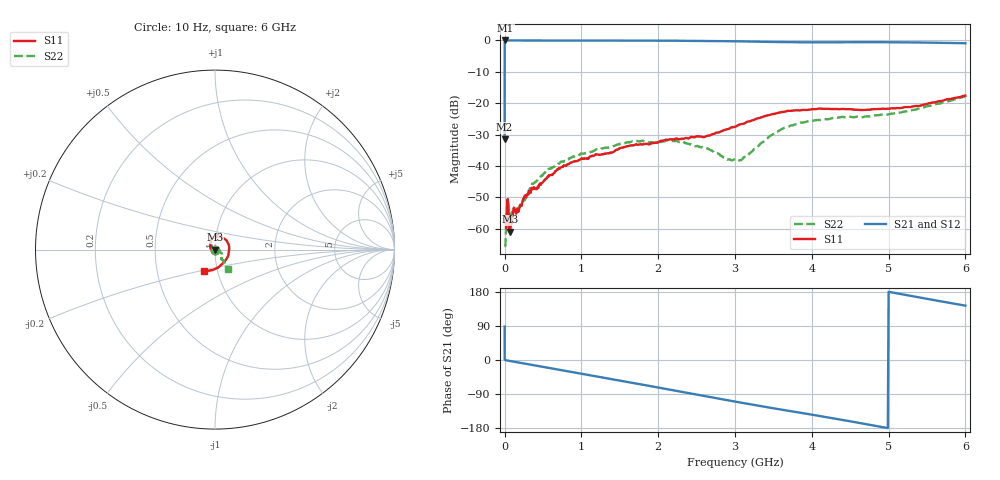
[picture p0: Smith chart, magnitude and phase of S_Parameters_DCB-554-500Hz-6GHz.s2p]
! MTS Systemtechnik GmbH
! S-Parameters
! Model: DCB-554-500Hz-6GHz
! Rohde & Schwarz ZVB8 2Ports - Version 3.20 - 1145.1010k08 SN: 100119
! Date: 2014-11-26 09:12:30
! S2P File: Measurements:
! <S11 S21 S12 S22>:
# HZ  S  DB  R  50.00
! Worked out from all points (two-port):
!   803 points, 10 Hz to 6 GHz, reference 50 ohm
!   highest |S21| = 0.00 dB at 10 MHz (marker M1); lowest = -31.5 dB at 10 Hz (marker M2)
!   |S21| within 3 dB of the highest: 428.2 Hz to end of sweep
!   lowest |S11| = -61.0 dB at 70 MHz (marker M3), VSWR 1.00, Z = 50.1 - j0.0502 ohm
!   |S11| at or under -10 dB: start of sweep to end of sweep
!   |S22| runs from -65.6 to -17.8 dB; largest |S21 - S12| = 0.0015
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10  -57.24 -121.5  -31.52 88.3  -31.52 88.3  -65.61 -123.6
260  -57.24 -121.5  -5.21 52.9  -5.21 52.9  -65.61 -123.6
310  -57.24 -121.5  -4.35 48.2  -4.35 48.2  -65.61 -123.6
810  -57.24 -121.5  -1.54 22.4  -1.54 22.4  -65.61 -123.6
1510  -57.24 -121.5  -0.96 13.1  -0.96 13.1  -65.61 -123.6
2960  -57.24 -121.5  -0.76 6.9  -0.76 6.9  -65.61 -123.6
10000  -57.24 -121.5  -0.61 1.6  -0.61 1.6  -65.61 -123.6
1000000  -57.24 -121.5  -0.61 1.6  -0.61 1.6  -65.61 -123.6
1e7  -57.24 -121.5  -0.00 -0.4  -0.00 -0.4  -65.61 -123.6
7e7  -61.00 -34.2  -0.00 -2.6  -0.00 -2.6  -56.90 -35.9
1e8  -56.95 -42.7  -0.01 -3.7  -0.01 -3.7  -54.84 -35.0
2.8e8  -50.01 -53.6  -0.01 -10.2  -0.02 -10.2  -50.01 -47.4
5.5e8  -43.93 -103.5  -0.02 -20.0  -0.03 -20.0  -41.22 -67.4
1.01e9  -37.74 -133.0  -0.03 -36.5  -0.03 -36.6  -36.10 -83.9
1.62e9  -33.66 -176.1  -0.05 -58.8  -0.05 -58.7  -32.53 -97.7
2.01e9  -32.38 162.9  -0.07 -73.0  -0.07 -73.0  -32.41 -102.3
2.33e9  -31.32 149.3  -0.10 -84.9  -0.10 -84.8  -32.41 -103.1
3.01e9  -27.43 128.1  -0.26 -110.1  -0.26 -110.1  -38.36 -64.5
3.61e9  -22.82 85.9  -0.53 -131.1  -0.53 -131.2  -28.24 -27.3
4.01e9  -21.87 49.7  -0.60 -144.5  -0.60 -144.6  -25.64 -40.8
5.01e9  -21.74 -36.2  -0.57 179.6  -0.57 179.6  -23.50 -55.5
6e9  -17.57 -116.3  -0.90 143.4  -0.90 143.4  -17.79 -56.2
